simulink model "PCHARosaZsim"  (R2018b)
settings: Solver=ode5  StartTime=0.0  StopTime=10  FixedStep=0.01  RelTol=1e-3  AbsTol=1e-6

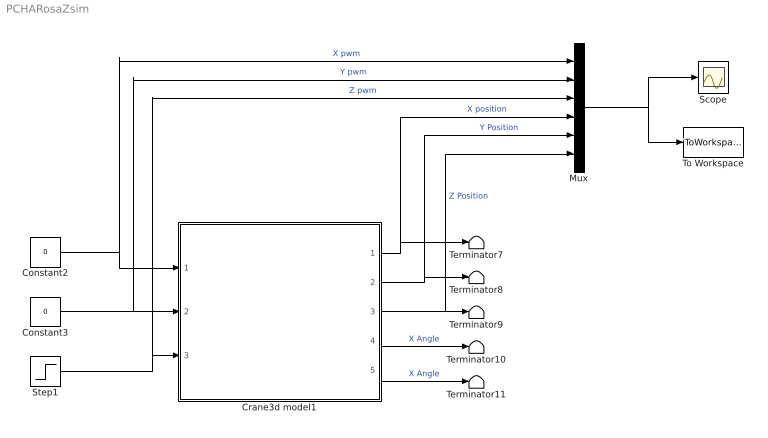
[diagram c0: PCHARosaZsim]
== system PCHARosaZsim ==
  Constant2 : Constant  Value=0
  Constant3 : Constant  Value=0
  Crane3d model1 : Subsystem  mask{RR=off, x0=[ 0.5, 0, 0,  0, 0, 0, 0, 0,  0.5, 0, -1]}
      mask prompts: RR "Model with constant length"; x0 "Initial conditions:[x,x',y,y',alfa,alfa',beta,beta',z,z',t]"
  Mux : Mux  Inputs=6
  Scope : Scope
  Step1 : Step  Time=0  After=-1  SampleTime=0.01
  Terminator{7..11} (5 alike) : Terminator
  To Workspace : ToWorkspace  VariableName=simout  SaveFormat=Timeseries  SampleTime=-1
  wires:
  Constant3/1 -> Crane3d model1/2(Y PWM), Mux/2  "Y pwm"
  Step1/1 -> Crane3d model1/3(Z PWM), Mux/3  "Z pwm"
  Constant2/1 -> Crane3d model1/1(X PWM), Mux/1  "X pwm"
  Mux/1 -> To Workspace/1, Scope/1
  Crane3d model1/1(X Posiion) -> Mux/4, Terminator7/1  "X position"
  Crane3d model1/2(Y Position) -> Mux/5, Terminator8/1  "Y Position"
  Crane3d model1/5(Y Angle) -> Terminator11/1  "X Angle"
  Crane3d model1/4(X Angle) -> Terminator10/1  "X Angle"
  Crane3d model1/3(Z Position) -> Mux/6, Terminator9/1  "Z Position"

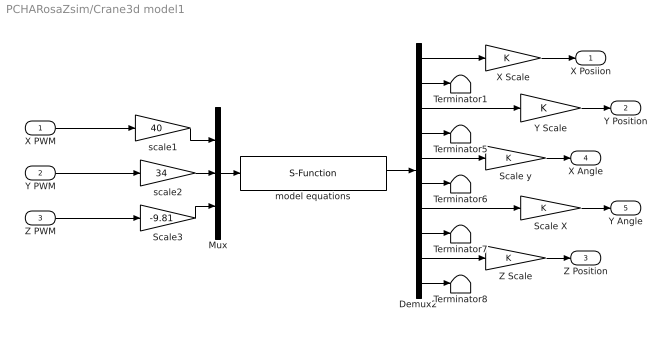
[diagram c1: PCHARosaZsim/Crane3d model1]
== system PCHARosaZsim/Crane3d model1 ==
  X PWM : Inport
  Y PWM : Inport  Port=2
  Z PWM : Inport  Port=3
  Demux2 : Demux  Outputs=10
  Mux : Mux  Inputs=3
  Scale X : Gain
  Scale y : Gain
  Scale3 : Gain  Gain=-9.81
  Terminator{1,5..8} (5 alike) : Terminator
  X Scale : Gain
  Y Scale : Gain
  Z Scale : Gain
  model equations : S-Function  FunctionName=model3dddm  Parameters=x0(1) x0(2) x0(3) x0(4) x0(5) x0(6) x0(7) x0(8) x0(9) x0(10) x0(11) RR  SFunctionDeploymentMode=off  EnableBusSupport=off
  scale1 : Gain  Gain=40
  scale2 : Gain  Gain=34
  X Posiion : Outport  Tag=X Position
  Y Position : Outport  Port=2
  Z Position : Outport  Port=3
  X Angle : Outport  Port=4
  Y Angle : Outport  Port=5
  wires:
  X PWM/1 -> scale1/1
  scale1/1 -> Mux/1
  Z PWM/1 -> Scale3/1
  Scale3/1 -> Mux/3
  Y PWM/1 -> scale2/1
  scale2/1 -> Mux/2
  Demux2/10 -> Terminator8/1
  Demux2/8 -> Terminator7/1
  Demux2/6 -> Terminator6/1
  Demux2/4 -> Terminator5/1
  Demux2/2 -> Terminator1/1
  Demux2/7 -> Scale X/1
  Scale X/1 -> Y Angle/1
  Demux2/5 -> Scale y/1
  Scale y/1 -> X Angle/1
  Demux2/9 -> Z Scale/1
  Z Scale/1 -> Z Position/1
  Demux2/3 -> Y Scale/1
  Demux2/1 -> X Scale/1
  X Scale/1 -> X Posiion/1
  model equations/1 -> Demux2/1
  Y Scale/1 -> Y Position/1
  Mux/1 -> model equations/1
